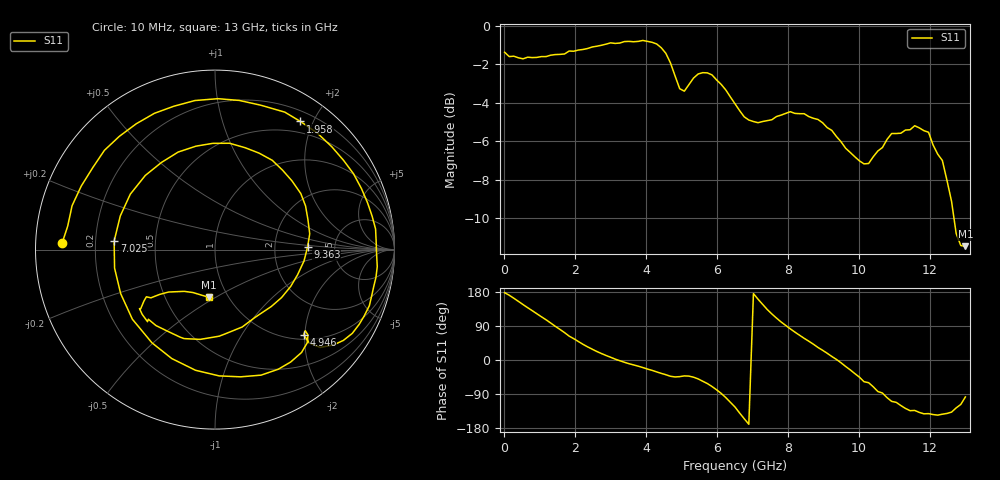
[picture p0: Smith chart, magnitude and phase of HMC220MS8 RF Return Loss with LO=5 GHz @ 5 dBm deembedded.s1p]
!Hittite Microwave Corporation
!12 Elizabeth Drive
!Chelmsford, MA 01824
!Tel: 978-250-3343
!Fax: 978-250-3373
!Device: HMC220MS8, 5-12 GHz, GaAS MMIC SMT Double-Balanced Mixer in 8-lead MSOP package
!Misc: RF Return Loss, LO = 5 GHz @ 5dBm, Room
# MHZ S MA R 50
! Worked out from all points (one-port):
!   101 points, 10 MHz to 13 GHz, reference 50 ohm
!   lowest |S11| = -11.4 dB at 13 GHz (marker M1), VSWR 1.73, Z = 40.7 - j23.3 ohm
!   |S11| at or under -10 dB: 12.68 GHz to end of sweep
!   S11 on the Smith chart (normalised r, x): 10 MHz: 0.08, +0.02; 1.958 GHz: 0.34, +1.82; 4.946 GHz: 1.10, -1.97; 7.025 GHz: 0.28, +0.04; 9.363 GHz: 3.13, +0.12; 13 GHz: 0.81, -0.47
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10  0.853 177.7
399.7  0.825 154.7
919.3  0.827 122.0
1309  0.838 97.7
1698.7  0.844 72.4
1958.5  0.858 56.3
2608  0.884 22.5
3257.5  0.901 -1.9
3907  0.915 -19.9
4426.6  0.876 -35.3
4946.2  0.686 -43.9
5335.9  0.731 -45.4
5725.6  0.754 -62.2
6115.3  0.704 -88.1
6505  0.627 -124.1
6764.8  0.58 -155.0
7024.6  0.564 175.1
7414.3  0.567 133.2
7674.1  0.581 110.6
8193.7  0.592 73.6
8843.2  0.571 33.1
9362.8  0.516 1.6
9752.5  0.469 -26.0
10791.7  0.507 -99.4
11441.2  0.537 -133.7
12350.5  0.447 -143.1
12740.2  0.289 -126.4
13000  0.268 -97.5
